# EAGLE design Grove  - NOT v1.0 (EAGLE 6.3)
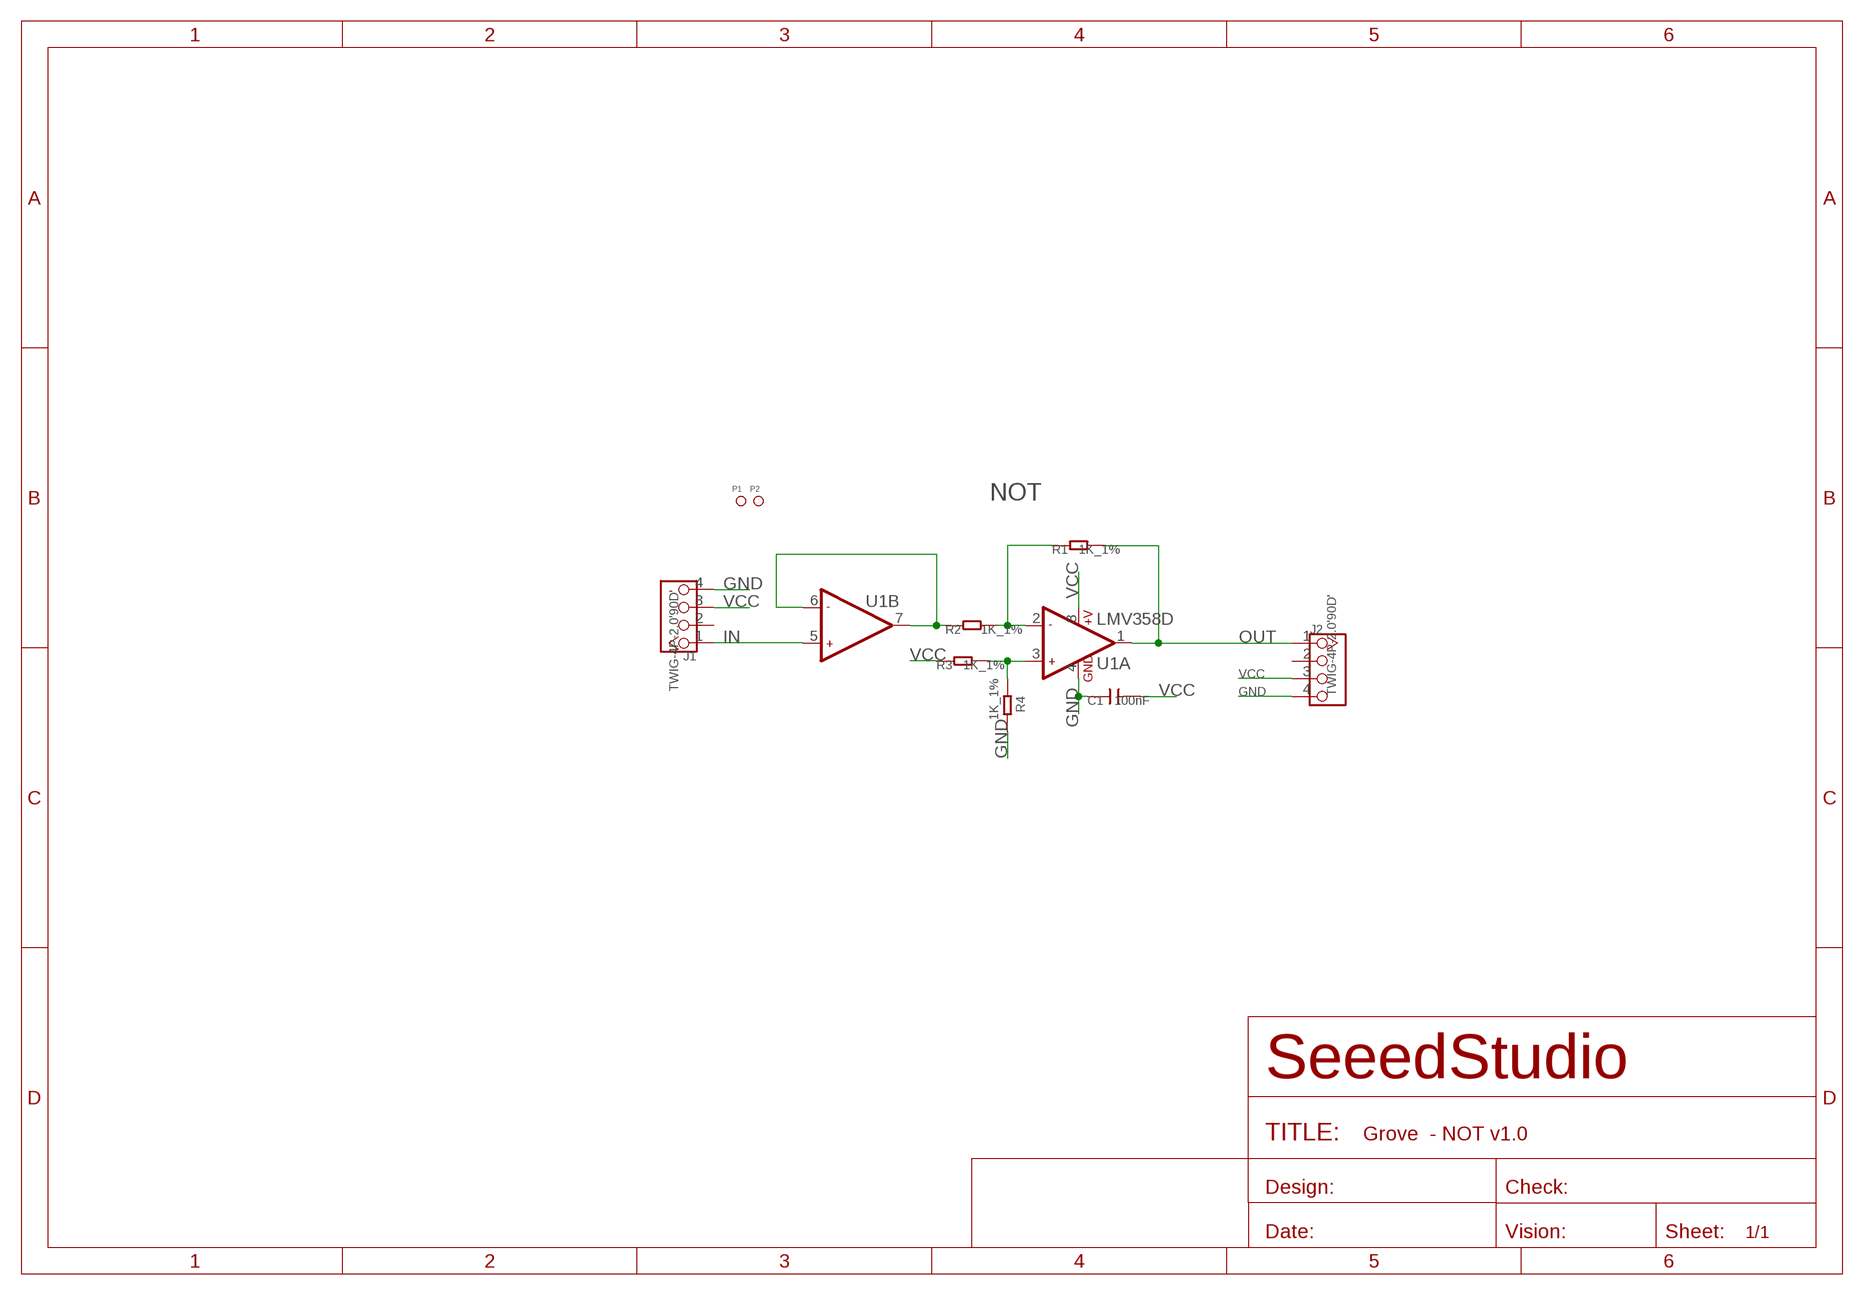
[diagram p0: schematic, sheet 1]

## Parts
C1  100nF  C-0603  [C0603]
J1  TWIG-4P-2.0'90D'  [4P-2.0-90D]
J2  TWIG-4P-2.0'90D'  [4P-2.0-90D]
P1  PAD-MARK  [ROUND-MARK-1.0]
P2  PAD-MARK  [ROUND-MARK-1.0]
R1  1K_1%  R-0603  [R0603]
R2  1K_1%  R-0603  [R0603]
R3  1K_1%  R-0603  [R0603]
R4  1K_1%  R-0603  [R0603]
U1  LMV358D  [SO08]

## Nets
GND: C1.1 J1.4 J2.4 R4.2 U1.4(A:GND)
IN: J1.1 U1.5(B:+IN2)
N$1: R3.2 R4.1 U1.3(A:+IN1)
N$2: R1.1 R2.2 U1.2(A:-IN1)
N$7: R2.1 U1.6(B:-IN2) U1.7(B:OUT2)
OUT: J2.1 R1.2 U1.1(A:OUT1)
VCC: C1.2 J1.3 J2.3 R3.1 U1.8(A:+V)
Unconnected: J1.2 J2.2

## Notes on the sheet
- NOT

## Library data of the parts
C1 = Discrete:C*: Ceramic Capacitors
J1 J2 = Connector:TWIG-4P-2.0
P1 P2 = Discrete:PAD-MARK; PARTNO: DNP
R1-R4 = Discrete:R*
U1 = IC:LMV358: General purpose LOW Voltage, Rail-to-Rail Output Amplifiers http://www.fairchildsemi.com/ds/LM/LMV358.pdf

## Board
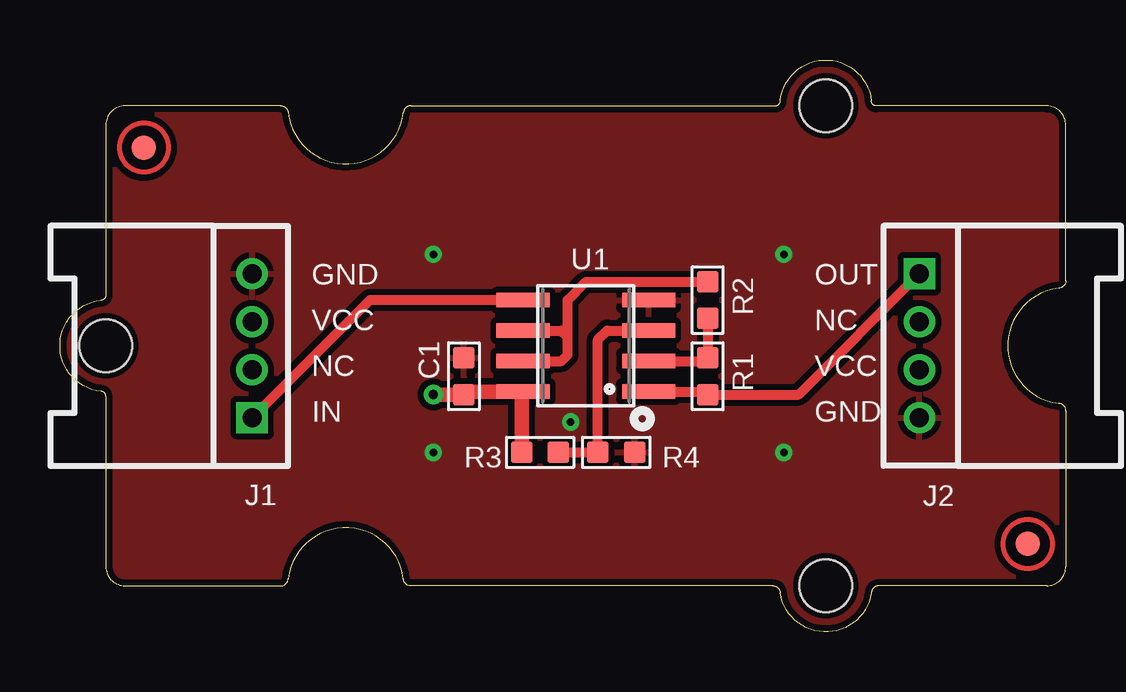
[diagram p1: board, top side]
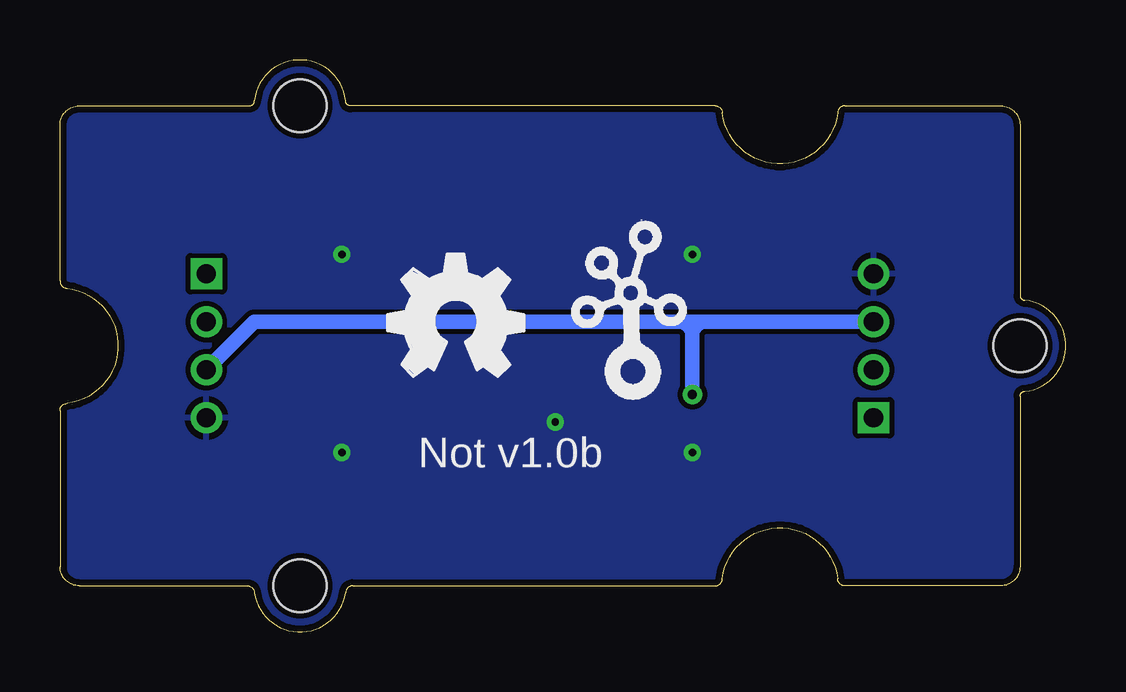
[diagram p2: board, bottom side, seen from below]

Size 41.91 x 23.83 mm. Coordinates in mm from the lower left corner, seen from the top.
Copper layers (1*16): Top 0.035mm / dielectric 1.5mm / Bottom 0.035mm
Design rules "default": minimum track width 10mil, minimum drill 12mil, track to track 8mil, track to pad 8mil, pad to pad 8mil, via to via 8mil, smd to smd 8mil, copper to edge 10mil, drill to drill 8mil, minimum pad ring 10mil, minimum via ring 8mil, stop-mask expansion 4mil, vias tented up to drill 25mil, thermal gap 10mil

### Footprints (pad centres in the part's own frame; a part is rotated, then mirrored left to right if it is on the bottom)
C0603 = smd 0.889 x 0.889: 1 -0.762,0; 2 0.762,0
4P-2.0-90D = drill 0.8 pad 1.27 square: 1 -3,0 | drill 0.8 pad 1.27: 2 -1,0; 3 1,0; 4 3,0
ROUND-MARK-1.0 = smd 1.016 x 1.016: P$1 0,0
R0603 = smd 0.889 x 0.889: 1 -0.762,0; 2 0.762,0
SO08 = smd 0.61 x 2.21: 1 -1.905,-2.616; 2 -0.635,-2.616; 3 0.635,-2.616; 4 1.905,-2.616; 5 1.905,2.616; 6 0.635,2.616; 7 -0.635,2.616; 8 -1.905,2.616
2U-DIM-W/DRILL = hole 2.2: -10,-10; -10,10; 20,0

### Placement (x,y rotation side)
C1  16.83,10.65 270 top
J1  8.01,11.92 90 top
J2  35.81,11.92 270 top
P1  40.32,3.67 0 top
P2  3.49,20.18 0 top
R1  26.99,10.65 270 top
R2  26.99,13.83 270 top
R3  20,7.48 0 top
R4  23.18,7.48 0 top
U1  21.91,11.92 90 top
U$2  [2U-DIM-W/DRILL]  21.91,11.92 180 top
U$3  [OSHW_FILLX200_NOTEXT]  28.26,10.65 0 bottom
U$4  [TWIGLOGO]  18.1,10.65 0 bottom

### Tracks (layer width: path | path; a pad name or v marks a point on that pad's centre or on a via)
GND  (via drill 0.3 pad 0.64)
  other vias: 15.56,15.73 15.56,7.48 30.16,7.48 30.16,15.73 21.27,8.75
  pour Bottom: 31.43,-0.14 42.23,-0.14 42.23,23.99 -0.32,23.99 -0.32,1.13 -0.32,-0.14 31.31,-0.14
  pour Top (isolate 0.254): 31.43,-0.14 42.23,-0.14 42.23,23.99 -0.32,23.99 -0.32,1.13 -0.32,-0.14 31.31,-0.14
IN
  Top 0.406: U1.5 12.91,13.83 J1.1
N$1
  Top 0.406: R3.2 R4.1 22.42,12.18 22.8,12.56 U1.3
N$2
  Top 0.406: U1.2 26.86,11.29 R1.1 R2.2
N$7
  Top 0.406: U1.6 20.89,12.56 | 20.89,12.56 21.02,12.56 21.15,12.68 | U1.7 20.89,11.29 21.15,11.54 21.15,12.3 | 21.15,12.3 21.15,12.68 | 21.15,12.3 20.89,12.56 | 26.86,14.72 R2.1 21.91,14.59 21.15,13.83 21.15,12.68
OUT
  Top 0.406: U1.1 26.86,10.02 R1.2 30.78,9.89 J2.1
VCC  (via drill 0.38 pad 0.81)
  Top 0.61: R3.1 19.24,9.97 U1.8 16.96,10.02 C1.2 v15.56,9.89
  Bottom 0.61: J1.3 15.69,12.92 | 15.69,12.92 33.81,12.92 J2.3 | v15.56,9.89 15.56,12.43 15.56,12.56 | 15.56,12.56 15.56,12.79 15.69,12.92 | 15.56,12.56 15.3,12.81 | 15.56,12.56 15.81,12.81

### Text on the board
tPlace: GND | OUT | VCC | NC | NC | VCC | IN | GND
bPlace: Not v1.0b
